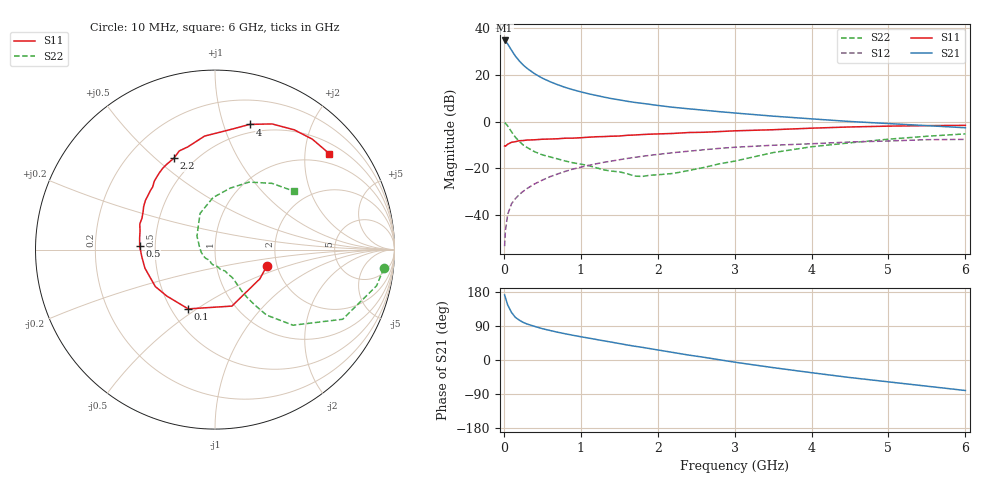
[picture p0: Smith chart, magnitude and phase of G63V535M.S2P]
! SIEMENS Small Signal Semiconductors
! BFG193
! Si NPN RF Bipolar Junction Transistor in SOT223
! VCE = 3.5 V  IC = 35 mA
! Common Emitter S-Parameters:  August  1996
# GHz  S  MA  R  50
!  f  S11  S21  S12  S22
! GHz  MAG  ANG  MAG  ANG  MAG  ANG  MAG  ANG
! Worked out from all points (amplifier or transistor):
!   36 points, 10 MHz to 6 GHz, reference 50 ohm
!   highest |S21| = 34.6 dB at 10 MHz (marker M1)
!   |S21| within 3 dB of that: start of sweep to 78.19 MHz
!   unconditionally stable (mu >= 1): 519.6 MHz to 2.345 GHz
!   at 250 MHz: K = 0.87, MSG = 27.0 dB, |S12| = -29.8 dB
!   at 1.4 GHz: K = 1.05, MAG = 12.0 dB, |S12| = -16.8 dB
!   at 6 GHz: K = 0.90, MSG = 2.5 dB, |S12| = -7.6 dB
!   S11 on the Smith chart (normalised r, x): 10 MHz: 1.77, -0.35; 100 MHz: 0.61, -0.46; 500 MHz: 0.41, +0.02; 2.2 GHz: 0.39, +0.58; 4 GHz: 0.42, +1.23; 6 GHz: 0.74, +2.56
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0.01  0.3033 -17.1  53.83 171.8  0.0022 86.7  0.9463 -6.3
0.02  0.2983 -33.0  52.23 164.9  0.0046 76.9  0.9226 -12.6
0.05  0.3286 -73.3  45.35 145.1  0.0105 73.7  0.8105 -28.6
0.1  0.3624 -114.3  33.31 125.4  0.0177 66.3  0.6053 -44.1
0.15  0.3727 -135.9  24.9 112.5  0.0227 62.9  0.4644 -51.8
0.2  0.3911 -148.2  19.78 105.2  0.0277 64.8  0.3811 -54.3
0.25  0.394 -157.7  16.22 99.4  0.0324 65.5  0.3182 -56.2
0.3  0.4039 -165.2  13.76 95.1  0.0372 66.1  0.2814 -57.1
0.4  0.4094 -174.1  10.5 88.7  0.0469 66.6  0.2275 -57.6
0.5  0.4202 177.5  8.447 82.7  0.0564 66.0  0.1956 -57.7
0.6  0.4247 171.4  7.109 77.9  0.0667 65.7  0.1764 -58.9
0.8  0.4426 161.2  5.349 69.1  0.0869 62.7  0.1441 -63.1
1.1  0.4645 148.8  3.928 57.9  0.1161 57.9  0.1151 -74.3
1.3  0.4793 141.6  3.337 50.6  0.1354 54.0  0.0934 -83.3
1.6  0.5094 131.6  2.719 39.8  0.1634 47.4  0.0777 -106.3
2.2  0.5586 114.2  2.019 19.9  0.2172 34.1  0.0783 -169.0
2.8  0.6127 99.6  1.631 0.7  0.2682 20.2  0.1255 143.2
3.5  0.6709 83.4  1.307 -20.1  0.3129 3.0  0.2182 112.4
4  0.7239 74.5  1.144 -33.5  0.3369 -6.8  0.2905 92.1
4.5  0.7688 65.6  1.005 -46.3  0.3669 -16.8  0.3528 76.1
5.5  0.8201 48.6  0.82 -69.1  0.4117 -40.1  0.4868 49.3
6  0.8314 40.0  0.739 -80.5  0.4172 -53.5  0.5471 36.5
